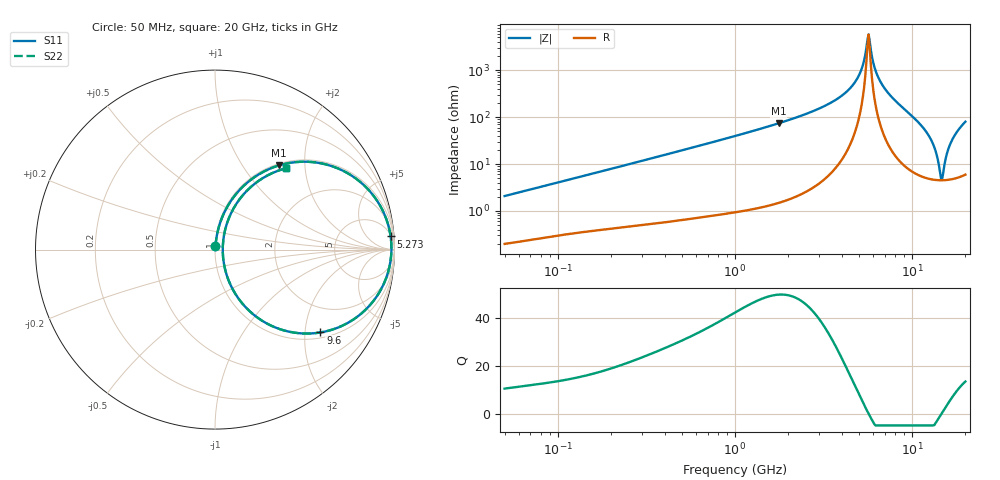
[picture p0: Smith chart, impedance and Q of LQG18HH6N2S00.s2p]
!Murata Part Number: LQG18HH6N2S00
!These Parameters are Measured in Series Mode Connection
!  o--[Z]--o
!Port1  Port2
!  o-------o
!Freq. Start=50[MHz] Stop=20[GHz], 401[Steps]
# Hz S RI R 50
!Freq.(Hz) S11(Real) S11(Imag) S21(Real) S21(Imag) S12(Real) S12(Imag) S22(Real) S22(Imag)
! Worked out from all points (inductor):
!   401 points, 50 MHz to 20 GHz, reference 50 ohm
!   read as one part in series: L = 6.54 nH near 51.52 MHz
!   highest Q = 49.8 at 1.767 GHz (marker M1), where L = 6.67 nH
!   self-resonance near 5.599 GHz
!   S11 on the Smith chart (normalised r, x): 50 MHz: 1.00, +0.04; 5.273 GHz: 6, +25; 9.6 GHz: 1.15, -2.41; 20 GHz: 1.12, +1.59
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5e7  0.0024 0.0206  0.9976 -0.0206  0.9976 -0.0206  0.0024 0.0206
1.364002e8  0.00643 0.0539  0.9936 -0.0539  0.9936 -0.0539  0.00643 0.0539
3.721004e8  0.0259 0.1409  0.9741 -0.1409  0.9741 -0.1409  0.0259 0.1409
1e9  0.1409 0.3363  0.8591 -0.3363  0.8591 -0.3363  0.1409 0.3363
1.766834e9  0.3567 0.4691  0.6433 -0.4691  0.6433 -0.4691  0.3567 0.4691
2.728004e9  0.6315 0.471  0.3685 -0.471  0.3685 -0.471  0.6315 0.471
4.275624e9  0.9131 0.2564  0.0869 -0.2564  0.0869 -0.2564  0.9131 0.2564
4.89267e9  0.9631 0.1438  0.0369 -0.1438  0.0369 -0.1438  0.9631 0.1438
5.273168e9  0.9785 0.0733  0.0215 -0.0733  0.0215 -0.0733  0.9785 0.0733
5.515528e9  0.9826 0.0288  0.0174 -0.0288  0.0174 -0.0288  0.9826 0.0288
5.683258e9  0.9831 -0.00159  0.0169 0.00159  0.0169 0.00159  0.9831 -0.00159
6.406762e9  0.964 -0.1271  0.036 0.1271  0.036 0.1271  0.964 -0.1271
7.442007e9  0.8855 -0.2824  0.1145 0.2824  0.1145 0.2824  0.8855 -0.2824
9.600142e9  0.5877 -0.4615  0.4123 0.4615  0.4123 0.4615  0.5877 -0.4615
1.098561e10  0.3622 -0.4435  0.6378 0.4435  0.6378 0.4435  0.3622 -0.4435
1.257102e10  0.1514 -0.2994  0.8486 0.2994  0.8486 0.2994  0.1514 -0.2994
1.354865e10  0.0739 -0.1669  0.9261 0.1669  0.9261 0.1669  0.0739 -0.1669
1.460232e10  0.0433 -0.0123  0.9567 0.0123  0.9567 0.0123  0.0433 -0.0123
1.504638e10  0.046 0.0513  0.954 -0.0513  0.954 -0.0513  0.046 0.0513
1.573793e10  0.066 0.1442  0.934 -0.1442  0.934 -0.1442  0.066 0.1442
1.670968e10  0.1199 0.2565  0.8801 -0.2565  0.8801 -0.2565  0.1199 0.2565
2e10  0.3973 0.4535  0.6027 -0.4535  0.6027 -0.4535  0.3973 0.4535
